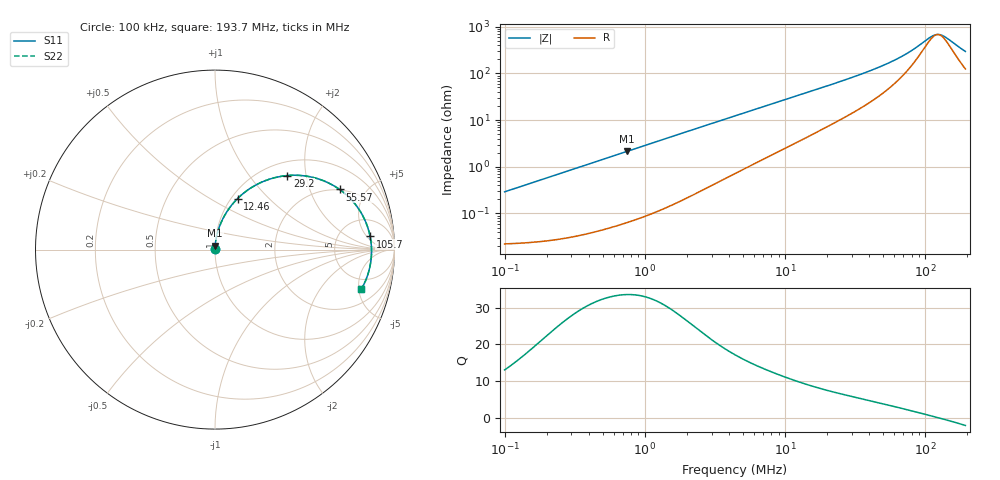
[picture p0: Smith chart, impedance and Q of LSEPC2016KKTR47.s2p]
! LSEPC2016KKTR47  S-PARAMETER MODEL  ( General Type )
! Model Generated by TAIYO YUDEN Corporation (http://www.ty-top.com)
! Version 1.0
! TAIYO YUDEN Control No. 180907NI43SB-FBB
! Copyright(c) 2018 TAIYO YUDEN CO.,LTD. All Rights Reserved.
! Product Description (link to TY-COMPAS)
! https://ds.yuden.co.jp/TYCOMPAS/or/detail?pn=LSEPC2016KKTR47M&u=M
! Products Name : Inductors
! Characteristics :
!  Inductance : 0.47 uH , SRF(min) : -Hz , DC Resistance(max) : 0.026 Ohm
!  Rated Current : Saturation :5300 mA , Temp Rise : 4700 mA (40 degC)
!  Case Size : 2.0 x 1.6 / 0.079 x 0.063 [mm/inch] , Thickness : 1 / 0.039 [mm/inch]
!  (Conditions: Temperature = 25 degC , DC Bias Current/Voltage = 0A / 0V)
! External Node Assignments :
!  1  o---GGG---o  2
! GND o---------o GND
! Frequency Range : 0.1MHz  -  193.730505MHz  [ 402 STEP ]
# MHz S RI R 50
! Freq[MHz].  S11 Real  S11 Imag  S21 Real  S21 Imag  S12 Real  S12 Imag  S22 Real  S22 Imag
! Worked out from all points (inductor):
!   401 points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, 100 kHz to 193.7 MHz, reference 50 ohm
!   read as one part in series: L = 461 nH near 103.9 kHz
!   highest Q = 33.6 at 743.2 kHz (marker M1), where L = 456 nH
!   self-resonance near 122.9 MHz
!   S11 on the Smith chart (normalised r, x): 100 kHz: 1.00, +0.01; 12.46 MHz: 1.07, +0.67; 29.2 MHz: 1.27, +1.56; 55.57 MHz: 1.97, +3.26; 105.7 MHz: 10, +6; 193.7 MHz: 3.49, -5.36
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0.1  0.000231 0.0029  0.9998 -0.0029  0.9998 -0.0029  0.000231 0.0029
0.355309  0.00045 0.0102  0.9995 -0.0102  0.9995 -0.0102  0.00045 0.0102
0.743203  0.00109 0.0213  0.9989 -0.0213  0.9989 -0.0213  0.00109 0.0213
1.262442  0.00243 0.0358  0.9976 -0.0358  0.9976 -0.0358  0.00243 0.0358
2.494935  0.00788 0.0697  0.9921 -0.0697  0.9921 -0.0697  0.00788 0.0697
4.401483  0.0217 0.1193  0.9783 -0.1193  0.9783 -0.1193  0.0217 0.1193
7.913286  0.0597 0.2005  0.9403 -0.2005  0.9403 -0.2005  0.0597 0.2005
12.46203  0.126 0.2847  0.874 -0.2847  0.874 -0.2847  0.126 0.2847
15.63884  0.1784 0.3291  0.8216 -0.3291  0.8216 -0.3291  0.1784 0.3291
21.16862  0.2728 0.3812  0.7272 -0.3812  0.7272 -0.3812  0.2728 0.3812
29.20105  0.4025 0.4126  0.5975 -0.4126  0.5975 -0.4126  0.4025 0.4126
40.28139  0.5509 0.401  0.4491 -0.401  0.4491 -0.401  0.5509 0.401
55.56615  0.6942 0.3352  0.3058 -0.3352  0.3058 -0.3352  0.6942 0.3352
65.88284  0.7583 0.2794  0.2417 -0.2794  0.2417 -0.2794  0.7583 0.2794
76.65072  0.8048 0.2201  0.1952 -0.2201  0.1952 -0.2201  0.8048 0.2201
87.50688  0.836 0.1624  0.164 -0.1624  0.164 -0.1624  0.836 0.1624
105.7358  0.8642 0.0735  0.1358 -0.0735  0.1358 -0.0735  0.8642 0.0735
118.4487  0.8713 0.018  0.1287 -0.018  0.1287 -0.018  0.8713 0.018
130.2027  0.8717 -0.0287  0.1283 0.0287  0.1283 0.0287  0.8717 -0.0287
140.4404  0.8682 -0.0661  0.1318 0.0661  0.1318 0.0661  0.8682 -0.0661
176.2414  0.8377 -0.1758  0.1623 0.1758  0.1623 0.1758  0.8377 -0.1758
193.7305  0.8162 -0.2191  0.1838 0.2191  0.1838 0.2191  0.8162 -0.2191
